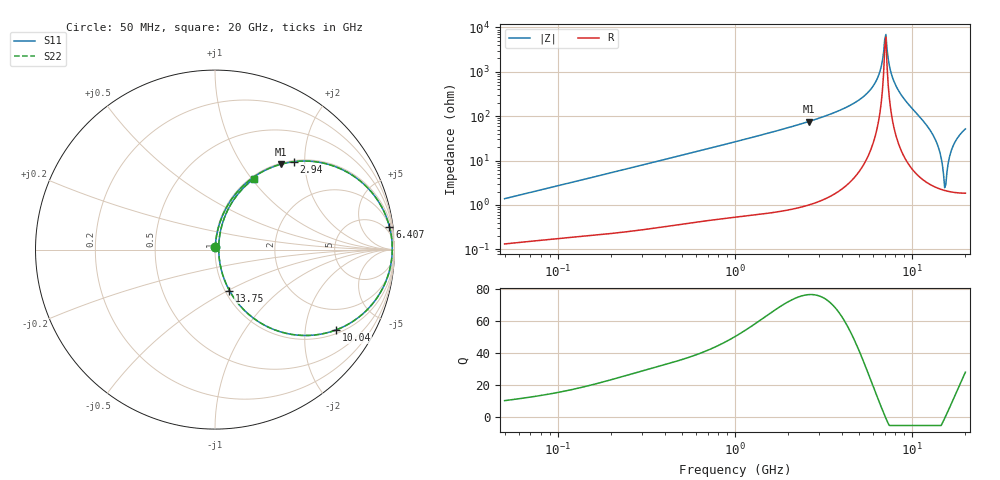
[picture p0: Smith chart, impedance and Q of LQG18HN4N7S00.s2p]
!Murata Part Number: LQG18HN4N7S00
!These Parameters are Measured in Series Mode Connection
!  o--[Z]--o
!Port1  Port2
!  o-------o
!Freq. Start=50[MHz] Stop=20[GHz], 401[Steps]
# Hz S RI R 50
!Freq.(Hz) S11(Real) S11(Imag) S21(Real) S21(Imag) S12(Real) S12(Imag) S22(Real) S22(Imag)
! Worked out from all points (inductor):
!   401 points, 50 MHz to 20 GHz, reference 50 ohm
!   read as one part in series: L = 4.34 nH near 51.52 MHz
!   highest Q = 76.3 at 2.608 GHz (marker M1), where L = 4.62 nH
!   self-resonance near 7.009 GHz
!   S11 on the Smith chart (normalised r, x): 50 MHz: 1.00, +0.03; 2.94 GHz: 1.02, +1.77; 6.407 GHz: 2, +15; 10.04 GHz: 1.13, -2.93; 13.75 GHz: 1.05, -0.51; 20 GHz: 1.04, +1.03
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5e7  0.0015 0.0137  0.9985 -0.0137  0.9985 -0.0137  0.0015 0.0137
1.364002e8  0.00327 0.0363  0.9967 -0.0363  0.9967 -0.0363  0.00327 0.0363
3.721004e8  0.0125 0.0966  0.9875 -0.0966  0.9875 -0.0966  0.0125 0.0966
1e9  0.0694 0.2444  0.9306 -0.2444  0.9306 -0.2444  0.0694 0.2444
2.608132e9  0.3663 0.4753  0.6337 -0.4753  0.6337 -0.4753  0.3663 0.4753
2.728004e9  0.3928 0.4819  0.6072 -0.4819  0.6072 -0.4819  0.3928 0.4819
2.940159e9  0.4398 0.4898  0.5602 -0.4898  0.5602 -0.4898  0.4398 0.4898
4.966507e9  0.8307 0.3634  0.1693 -0.3634  0.1693 -0.3634  0.8307 0.3634
5.769027e9  0.927 0.2407  0.073 -0.2407  0.073 -0.2407  0.927 0.2407
6.406762e9  0.9722 0.1273  0.0278 -0.1273  0.0278 -0.1273  0.9722 0.1273
7.009217e9  0.9876 0.0134  0.0124 -0.0134  0.0124 -0.0134  0.9876 0.0134
7.222371e9  0.9866 -0.0273  0.0134 0.0273  0.0134 0.0273  0.9866 -0.0273
7.442007e9  0.9819 -0.0692  0.0181 0.0692  0.0181 0.0692  0.9819 -0.0692
8.264682e9  0.9324 -0.2194  0.0676 0.2194  0.0676 0.2194  0.9324 -0.2194
1.004137e10  0.6761 -0.447  0.3239 0.447  0.3239 0.447  0.6761 -0.447
1.220001e10  0.2699 -0.4182  0.7301 0.4182  0.7301 0.4182  0.2699 -0.4182
1.375312e10  0.0805 -0.2282  0.9195 0.2282  0.9195 0.2282  0.0805 -0.2282
1.438523e10  0.0418 -0.137  0.9582 0.137  0.9582 0.137  0.0418 -0.137
1.504638e10  0.0229 -0.0429  0.9771 0.0429  0.9771 0.0429  0.0229 -0.0429
1.550395e10  0.0207 0.0189  0.9793 -0.0189  0.9793 -0.0189  0.0207 0.0189
1.696185e10  0.0564 0.1879  0.9436 -0.1879  0.9436 -0.1879  0.0564 0.1879
2e10  0.2184 0.3958  0.7816 -0.3958  0.7816 -0.3958  0.2184 0.3958
